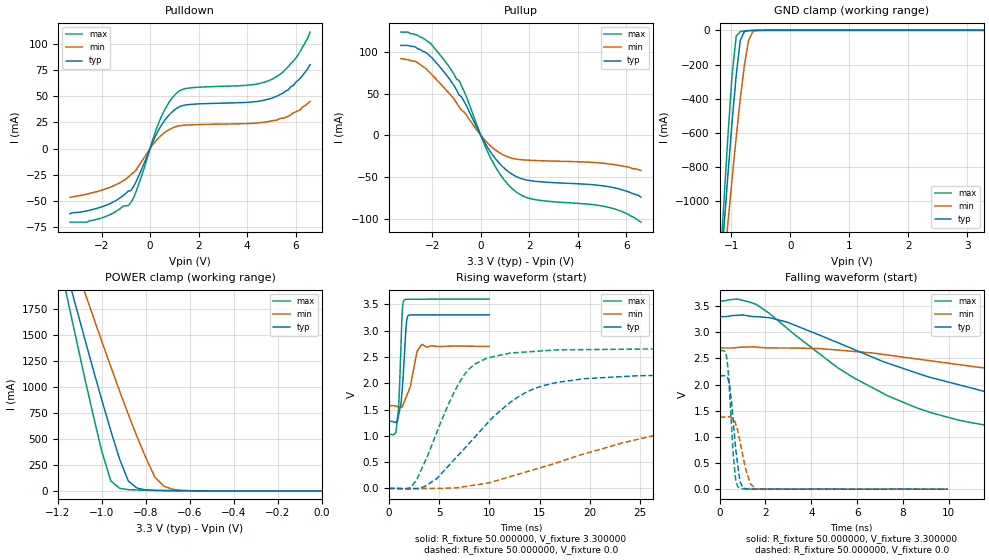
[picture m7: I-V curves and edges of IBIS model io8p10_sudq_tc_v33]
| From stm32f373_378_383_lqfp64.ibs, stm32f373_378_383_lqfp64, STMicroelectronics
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|   Model io8p10_sudq_tc_v33
[Model]  io8p10_sudq_tc_v33
Model_type I/O
Polarity   Non-Inverting
Enable   Active-Low
Vinl =   0.990000V
Vinh =   2.310000V
Vmeas =  1.650000V
Cref =   50.000000pF
Rref =   100.000000M
Vref =   0.0V
C_comp   1.325200pF   1.251200pF   1.426700pF
[Temperature Range]   25.000000   0.125000k   -40.000000
[Pullup Reference]   3.300000V   2.700000V   3.600000V
[Pulldown Reference]   0.0V   0.0V   0.0V
[POWER Clamp Reference]   3.300000V   2.700000V   3.600000V
[GND Clamp Reference]   0.0V   0.0V   0.0V
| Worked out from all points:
|   slope of the pulldown table from 0 to 0.495 V, typ, clamps not added: 21.3 ohm
|   slope of the pullup table from 0 to 0.495 V, typ, clamps not added: 20.9 ohm
|   GND clamp passes 1 mA (typ) near -0.67 V on its own axis
|   POWER clamp passes 1 mA (typ) near -0.60 V on its own axis
|   rising waveform, R_fixture 50.000000, V_fixture 3.300000: 20-80 % time 415ps typ, 825ps min, 303ps max; typ from 1.27 V to 3.3 V
|   rising waveform, R_fixture 50.000000, V_fixture 0.0: 20-80 % time 6.85ns typ, 16.4ns min, 3.72ns max; typ from 0 V to 2.17 V
|   falling waveform, R_fixture 50.000000, V_fixture 3.300000: 20-80 % time 9.34ns typ, 15.5ns min, 5.76ns max; typ from 3.3 V to 1.27 V
|   falling waveform, R_fixture 50.000000, V_fixture 0.0: 20-80 % time 298ps typ, 414ps min, 226ps max; typ from 2.17 V to 0 V
[Pulldown]
|Voltage   I(typ)   I(min)   I(max)
-3.3V     -62mA      -46.4mA    -70mA
-2V       -55.5mA    -39.6mA    -66mA
-800mV    -40.04mA   -24.89mA   -51.58mA
-500mV    -27.57mA   -17.6mA    -36.07mA
400mV     19.71mA    11.36mA    27.01mA
700mV     29.83mA    16.93mA    40.97mA
1.1V      38.46mA    21.2mA     53.02mA
1.6V      41.98mA    22.62mA    57.7mA
4.1V      44.26mA    24mA       60.59mA
5V        47.9mA     26.3mA     65.8mA
5.9V      60mA       34mA       83mA
6.6V      80mA       45mA       111mA
[Pullup]
|Voltage   I(typ)   I(min)   I(max)
-3.3V     108mA      92mA       124mA
-2.7V     106mA      89mA       121mA
-2.2V     98mA       78.2mA     113mA
-1.4V     71.8mA     53.5mA     86.1mA
-900mV    48.51mA    34.23mA    66.14mA
-700mV    41.33mA    28.36mA    53.31mA
400mV     -19.77mA   -12.52mA   -26.8mA
900mV     -37.48mA   -22.89mA   -50.99mA
1.4V      -48.39mA   -28.06mA   -66.43mA
2.2V      -54.79mA   -29.98mA   -76.75mA
5.3V      -61.6mA    -34.2mA    -86.4mA
6.6V      -74mA      -42mA      -104mA
[GND_clamp]
|Voltage   I(typ)   I(min)   I(max)
-3.3V     -9.739A    -9.975A    -9.587A
-1.2V     -1.489A    -1.65A     -1.416A
-1.13V    -1.162A    -1.385A    -1.009A
-1.06V    -842.2mA   -1.125A    -616.9mA
-990mV    -537.1mA   -870.1mA   -263mA
-920mV    -262.4mA   -625.3mA   -33.96mA
-850mV    -56.94mA   -397.4mA   -7.08mA
-780mV    -7.011mA   -202.2mA   -3.71mA
-710mV    -1.778mA   -58.23mA   -1.736mA
-640mV    -550uA     -8.783mA   -542.4uA
-570mV    -109.8uA   -1.292mA   -86.89uA
3.28V     0A         0A         0A
[POWER_clamp]
|Voltage   I(typ)   I(min)   I(max)
-3.28V    9.897A     9.838A     9.594A
-1.16V    2.103A     2.419A     1.88A
-1.12V    1.788A     2.17A      1.488A
-1.08V    1.476A     1.923A     1.102A
-1V       868.1mA    1.435A     373.1mA
-960mV    578.2mA    1.196A     96.06mA
-880mV    93.24mA    734.1mA    12.01mA
-840mV    26.3mA     517.4mA    8.56mA
-760mV    5.106mA    134mA      5.119mA
-720mV    3.355mA    46.34mA    3.808mA
-600mV    1.005mA    2.564mA    1.072mA
0V        0A         0A         0A
[Ramp]
| variable   typ   min   max
dV/dt_r  1.30032/6.84768n   0.81162/16.46324n   1.58898/3.71642n
dV/dt_f  1.21476/9.33495n   0.66960/15.56412n   1.54242/5.75707n
R_load = 50.000000
[Rising Waveform]
R_fixture= 50.000000
V_fixture= 3.300000
V_fixture_min= 2.700000
V_fixture_max= 3.600000
|time   V(typ)   V(min)   V(max)
0s        1.275V     1.571V     1.029V
720.7ps   1.266V     1.564V     1.094V
961ps     1.383V     1.552V     1.517V
1.201ns   1.603V     1.549V     2.685V
1.341ns   1.902V     1.554V     3.394V
1.502ns   2.382V     1.632V     3.578V
1.842ns   3.258V     1.795V     3.597V
2.803ns   3.299V     2.604V     3.596V
3.283ns   3.299V     2.738V     3.597V
9.97ns    3.3V       2.7V       3.6V
[Rising Waveform]
R_fixture= 50.000000
V_fixture= 0.0
V_fixture_min= 0.0
V_fixture_max= 0.0
|time   V(typ)   V(min)   V(max)
0s        1.051nV    9.611nV    1.582nV
2.302ns   -1.493mV   -3.505mV   46.07mV
4.705ns   179.9mV    23.66uV    1.034V
7.007ns   651.6mV    19.49mV    2.008V
8.008ns   862.1mV    48.77mV    2.275V
9.71ns    1.221V     98.54mV    2.475V
13.91ns   1.851V     328.3mV    2.597V
19.32ns   2.084V     651.6mV    2.639V
31.53ns   2.158V     1.172V     2.649V
49.85ns   2.167V     1.378V     2.648V
[Falling Waveform]
R_fixture= 50.000000
V_fixture= 3.300000
V_fixture_min= 2.700000
V_fixture_max= 3.600000
|time   V(typ)   V(min)   V(max)
0s        3.3V       2.7V       3.6V
1.602ns   3.298V     2.718V     3.532V
2.903ns   3.2V       2.699V     3.092V
5.105ns   2.811V     2.662V     2.337V
7.307ns   2.414V     2.567V     1.793V
9.309ns   2.125V     2.449V     1.452V
12.11ns   1.822V     2.29V      1.194V
19.72ns   1.407V     1.942V     1.052V
35.14ns   1.281V     1.626V     1.03V
49.85ns   1.275V     1.571V     1.029V
[Falling Waveform]
R_fixture= 50.000000
V_fixture= 0.0
V_fixture_min= 0.0
V_fixture_max= 0.0
|time   V(typ)   V(min)   V(max)
0s        2.167V     1.378V     2.648V
320.3ps   2.145V     1.382V     2.469V
440.4ps   1.956V     1.385V     1.781V
600.6ps   1.256V     1.342V     614mV
700.7ps   759.4mV    1.242V     169.4mV
840.8ps   287.3mV    1.01V      28.93mV
1.001ns   32.6mV     658.3mV    7.853mV
1.161ns   10.1mV     340.6mV    2.599mV
1.582ns   1.001mV    5.579mV    1.033mV
9.97ns    1.051nV    9.611nV    1.582nV
